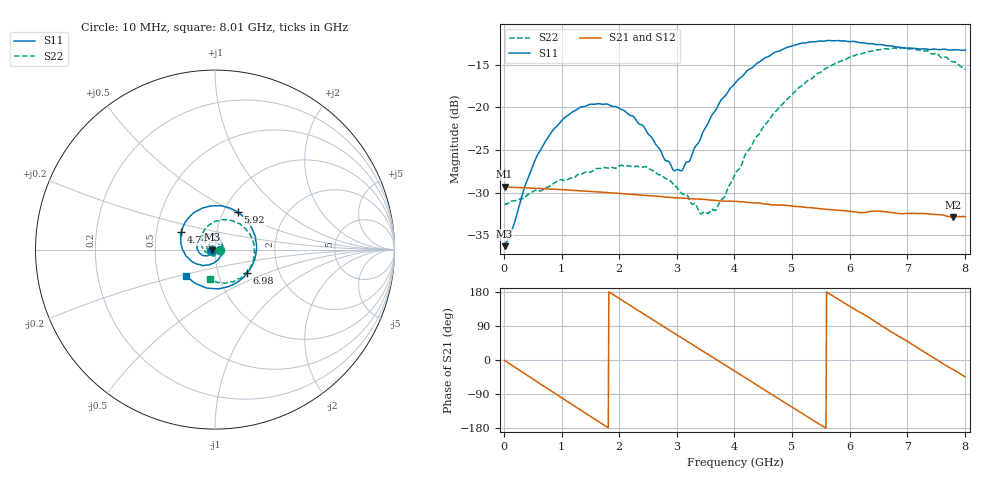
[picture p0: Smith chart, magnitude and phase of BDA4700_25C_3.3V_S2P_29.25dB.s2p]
!Agilent Technologies,E5071B,MY42404982,A.09.10
!Date: Mon Oct 20 18:15:22 2025
!Data & Calibration Information:
!Freq	S11:SOLT2(ON)	S21:SOLT2(ON)	S12:SOLT2(ON)	S22:SOLT2(ON)
# Hz S RI R 50
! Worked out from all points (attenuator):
!   801 points, 10 MHz to 8.01 GHz, reference 50 ohm
!   highest |S21| = -29.30 dB at 10 MHz (marker M1); lowest = -32.9 dB at 7.8 GHz (marker M2)
!   lowest |S11| = -36.3 dB at 10 MHz (marker M3), VSWR 1.03, Z = 48.5 - j0.115 ohm
!   |S11| at or under -10 dB: start of sweep to end of sweep
!   |S22| runs from -32.5 to -13.0 dB; largest |S21 - S12| = 0.00042
!   S11 on the Smith chart (normalised r, x): 10 MHz: 0.97, -0.00; 4.74 GHz: 0.67, +0.14; 5.92 GHz: 1.17, +0.52; 6.98 GHz: 1.37, -0.38; 8.01 GHz: 0.70, -0.21
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1e7  -0.0153 -0.00118  0.0343 -0.00071  0.0343 -0.000748  0.0272 -0.00076
1.4e8  -0.0166 -0.00975  0.033 -0.00839  0.033 -0.00844  0.0275 -0.00694
5.9e8  -0.041 -0.0342  0.0172 -0.0287  0.0172 -0.0287  0.0139 -0.0295
1e9  -0.0798 -0.0245  -0.00551 -0.0325  -0.00548 -0.0325  -0.0146 -0.0348
1.35e9  -0.1002 0.00936  -0.0226 -0.0233  -0.0226 -0.0233  -0.0365 -0.0183
2.07e9  -0.0482 0.0831  -0.0285 0.0128  -0.0284 0.0129  -0.031 0.0332
2.68e9  0.0322 0.0486  -0.00357 0.0299  -0.00365 0.0299  0.0127 0.0384
2.94e9  0.0422 0.00759  0.00908 0.0282  0.00911 0.0281  0.0253 0.0249
3.09e9  0.0385 -0.0184  0.0158 0.0248  0.0155 0.0249  0.0284 0.0129
3.41e9  0.00471 -0.0652  0.0258 0.0133  0.0258 0.0133  0.0213 -0.0108
3.55e9  -0.0193 -0.0793  0.0279 0.00694  0.0279 0.00688  0.0132 -0.02
3.69e9  -0.0475 -0.0859  0.0285 0.000361  0.0285 0.000246  0.00173 -0.0252
4.01e9  -0.1179 -0.0718  0.0244 -0.014  0.0245 -0.0139  -0.0309 -0.0259
4.74e9  -0.1883 0.0969  -0.00433 -0.0264  -0.00422 -0.0265  -0.0787 0.0557
5.35e9  -0.0621 0.2332  -0.0238 -0.00991  -0.0238 -0.01  -0.016 0.1467
5.92e9  0.1268 0.2092  -0.0213 0.0127  -0.0213 0.0126  0.1112 0.1545
6.35e9  0.2181 0.0879  -0.0087 0.023  -0.00863 0.0229  0.1945 0.0855
6.68e9  0.2263 -0.0325  0.00483 0.0239  0.00488 0.0238  0.219 0.00101
6.98e9  0.178 -0.1323  0.015 0.0187  0.015 0.0186  0.2063 -0.0794
7.43e9  0.034 -0.2157  0.0235 0.00358  0.0235 0.0035  0.1204 -0.1662
7.8e9  -0.1015 -0.1916  0.0206 -0.0098  0.0206 -0.00984  0.0207 -0.1836
8.01e9  -0.1611 -0.1445  0.0162 -0.0161  0.0163 -0.0162  -0.0294 -0.1636
